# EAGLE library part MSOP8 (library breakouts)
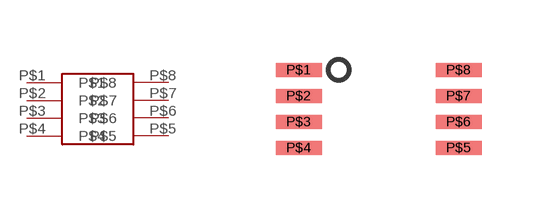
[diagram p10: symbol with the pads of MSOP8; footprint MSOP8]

Designator prefix -

## MSOP8  [MSOP8]
P$1  P$1
P$2  P$2
P$3  P$3
P$4  P$4
P$5  P$5
P$6  P$6
P$7  P$7
P$8  P$8

## Footprint MSOP8 (pad centres in mm)
smd 1.15 x 0.35: P$1 -2,0.975; P$2 -2,0.325; P$3 -2,-0.325; P$4 -2,-0.975; P$5 2,-0.975; P$6 2,-0.325; P$7 2,0.325; P$8 2,0.975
